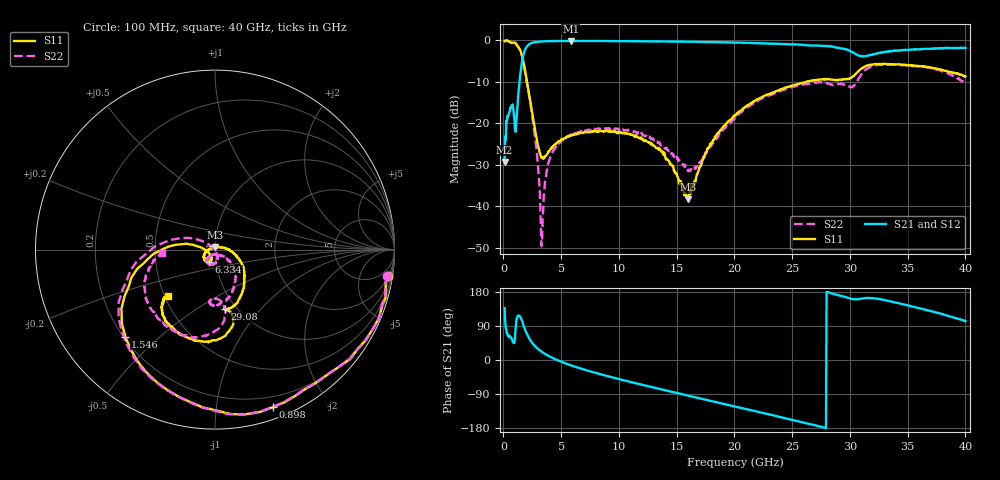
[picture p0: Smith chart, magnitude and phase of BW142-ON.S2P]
!  2-Port S-parameters saved by WinCal
! VAR MeasName=S-Parameters (CALIBRATED_DATA) read from VNA (N5244A)
! VAR MeasDate=11/21/2012 5:53:40 PM
! VAR NAME=128935
! VAR FILENAME=128935.S2P
! VAR DATE=11/21/2012 5:53:40 PM
! VAR PHYS_PORTS=1,2
# Hz S MA R 50
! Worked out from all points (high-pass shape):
!   801 points, 100 MHz to 40 GHz, reference 50 ohm
!   highest |S21| = -0.19 dB at 5.836 GHz (marker M1); lowest = -29.3 dB at 100 MHz (marker M2)
!   |S21| within 3 dB of the highest: 1.767 GHz to 30.41 GHz (28.64 GHz wide, 178 % of centre); 32.42 GHz to end of sweep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
!   lowest |S11| = -38.3 dB at 16.01 GHz (marker M3), VSWR 1.02, Z = 50 + j1.22 ohm
!   |S11| at or under -10 dB: 2.038 GHz to 26.27 GHz (24.23 GHz wide, 171 % of centre)
!   |S22| runs from -49.5 to -0.1 dB; largest |S21 - S12| = 0.016
!   S11 on the Smith chart (normalised r, x): 100 MHz: 2, -13; 898 MHz: 0.10, -1.43; 1.546 GHz: 0.21, -0.39; 6.334 GHz: 0.93, -0.12; 29.08 GHz: 0.88, -0.66; 40 GHz: 0.52, -0.31
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1e8  0.9744 -8.6  0.03425 136.7  0.03534 134.6  0.9708 -8.7
4.49125e8  0.968 -35.0  0.1272 65.1  0.1276 64.9  0.9688 -35.3
8.98e8  0.9354 -69.8  0.1302 44.7  0.1306 44.8  0.9344 -70.5
1.147375e9  0.8818 -94.4  0.1255 110.3  0.1253 109.9  0.8787 -95.8
1.546375e9  0.6964 -135.9  0.4778 108.0  0.4769 108.0  0.692 -138.7
2.095e9  0.2856 179.0  0.8572 64.6  0.8561 64.6  0.2774 170.9
2.79325e9  0.07476 172.0  0.9491 34.8  0.9483 34.8  0.05818 141.9
3.19225e9  0.04247 -162.9  0.9615 24.5  0.9617 24.4  0.009869 144.0
3.341875e9  0.03904 -149.0  0.9638 21.2  0.9641 21.1  0.003694 -105.8
4.040125e9  0.04848 -115.2  0.9735 8.4  0.9726 8.5  0.0381 -69.6
5.835625e9  0.07105 -113.6  0.9789 -14.0  0.9773 -14.0  0.07327 -86.2
6.334375e9  0.07483 -117.3  0.9781 -19.0  0.9769 -19.1  0.07675 -91.2
6.78325e9  0.07655 -119.3  0.9772 -23.4  0.9765 -23.3  0.07899 -94.2
1.341662e10  0.05062 -168.2  0.9633 -75.6  0.9629 -75.8  0.05888 -131.6
1.601012e10  0.01217 90.3  0.9581 -94.2  0.9573 -94.2  0.02644 -95.6
1.780562e10  0.05114 11.5  0.9494 -107.1  0.9495 -106.9  0.0495 -43.3
2.005e10  0.1256 -17.5  0.9318 -122.9  0.9362 -122.8  0.118 -39.3
2.673325e10  0.3277 -69.9  0.8599 -170.4  0.8602 -170.4  0.3033 -85.6
2.907738e10  0.3341 -80.7  0.8019 170.0  0.806 170.3  0.298 -95.0
3.097262e10  0.4504 -79.0  0.6428 161.7  0.6414 161.0  0.3826 -82.1
3.336662e10  0.5136 -105.8  0.7286 155.6  0.7376 155.1  0.5083 -115.0
4e10  0.367 -135.7  0.808 102.5  0.7963 103.1  0.2985 -176.0
